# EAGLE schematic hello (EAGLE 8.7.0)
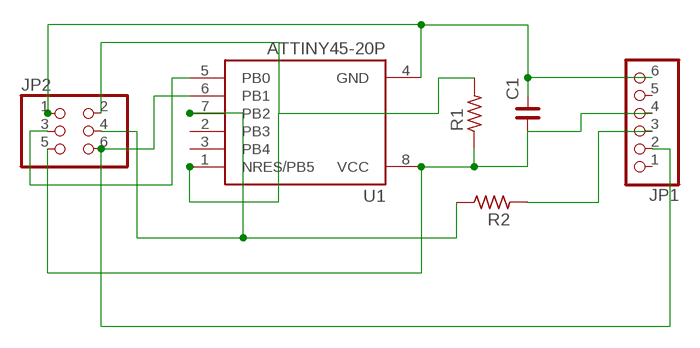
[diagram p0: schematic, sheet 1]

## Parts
C1  C_0805  [C0805]
JP1  PINHD-1X6  [1X06]
JP2  PINHD-2X3  [2X03]
R1  R_1005  [R1005]
R2  R_1005  [R1005]
U1  ATTINY45-20P  [PDIP08_300MIL]

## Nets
N$1: C1.2 JP1.6 JP2.1 U1.4(GND)
N$2: JP2.3 U1.5(PB0)
N$3: C1.1 JP1.4 JP2.5 R1.1 U1.8(VCC)
N$4: JP1.2 JP2.6 U1.6(PB1)
N$5: JP2.4 R2.2 U1.7(PB2)
N$6: JP2.2 R1.2 U1.1(NRES/PB5)
N$8: JP1.3 R2.1
Unconnected: JP1.1 JP1.5 U1.2(PB3) U1.3(PB4)

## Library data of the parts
C1 = rc-master-smd (1):C_: NON-POLARIZED CAP
JP1 = pinhead:PINHD-1X6: PIN HEADER
JP2 = pinhead:PINHD-2X3: PIN HEADER
R1 R2 = rc-master-smd (1):R_: RESISTOR
U1 = _hhn_attiny25_45_85:ATTINY45*: ATMEL ATtiny 45 Packages: P = PDIP 08 30mil S = SOIC 08 EIAJ 208mil X = TSSOP 08 4.4mm Technologies Note: for complete ordering code (temp. range, finish, tape&reel etc.) see www.atmel.com &bull; Supply Voltage: V = (1.8&hellip;5.5)V | [blank] = (2.7&hellip;5.5)V &bull; Speed: 10 = 10 MHz | 20 = 20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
